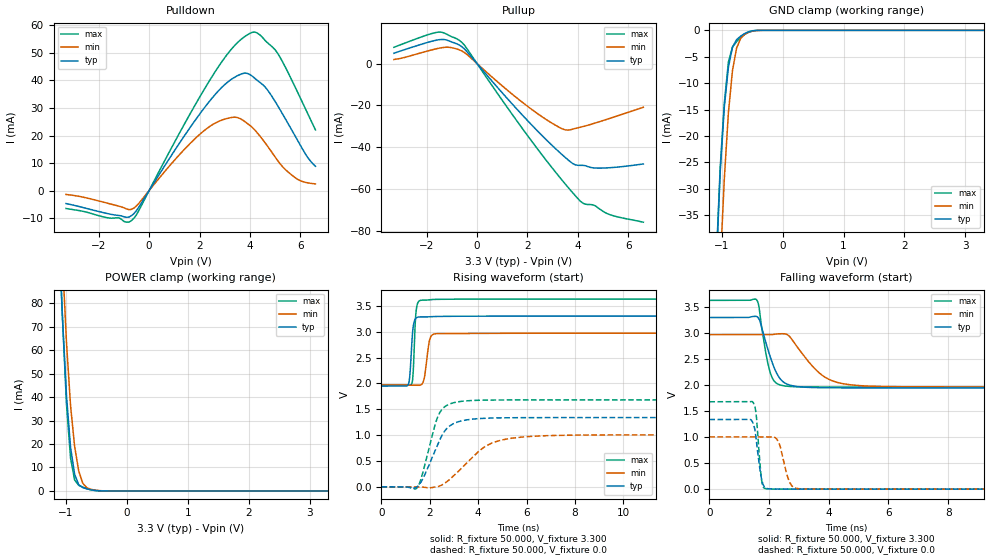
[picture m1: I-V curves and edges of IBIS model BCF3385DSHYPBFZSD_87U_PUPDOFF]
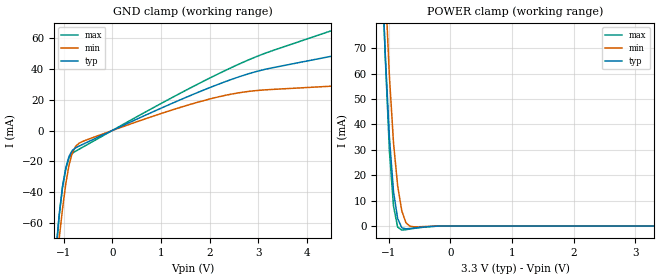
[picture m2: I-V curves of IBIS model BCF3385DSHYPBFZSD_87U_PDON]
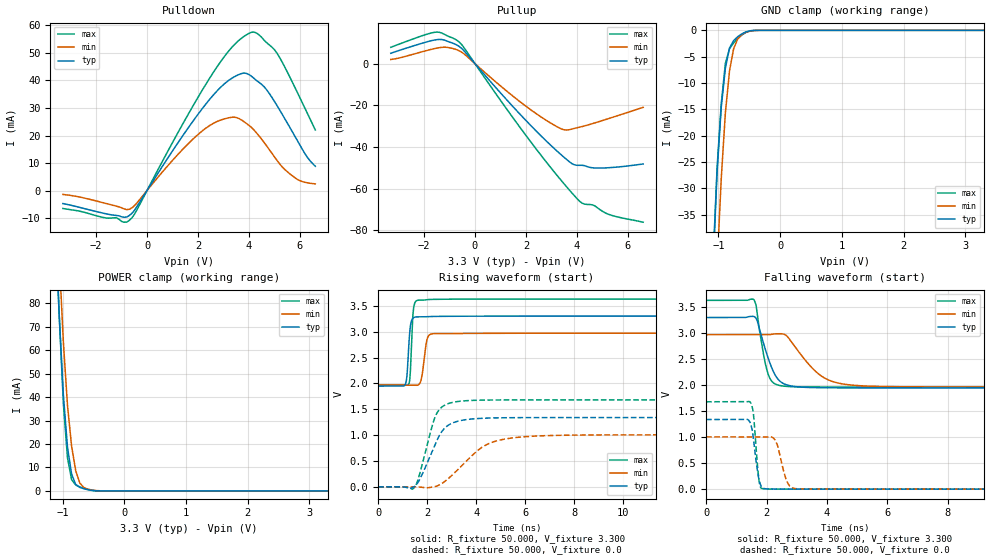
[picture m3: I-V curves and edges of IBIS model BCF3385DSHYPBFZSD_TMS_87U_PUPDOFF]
[IBIS VER]   5.0
[File Name]   am13e230pmg.ibs
[File Rev]   1.0
[Date]   February 08, 2026
[Source]   File originated at Texas Instruments
[Copyright]   (c) 2012, Texas Instruments Inc.
[Component]   am13e230pmg
[Manufacturer] Texas Instruments
[Package]
| Variable   Typ   Min   Max
   R_pkg 2.77E-01 1.56E-01 3.36E-01
   L_pkg 5.39E-09 4.33E-09 6.28E-09
   C_pkg 2.25E-14 1.68E-14 4.82E-14
[Pin]   signal_name   model_name   R_pin   L_pin   C_pin
   1   VDD   NC 3.29E-01 6.19E-09 4.32E-14
   2   PB13   BCF3385DSWHYPBFZSD_87U 3.06E-01 5.86E-09 2.08E-14
   3   PB14   BCF3385DSHYPBFZSD_87U 2.92E-01 5.63E-09 2.01E-14
   4   PB15   BCF3385DSHYPBFZSD_87U 2.81E-01 5.42E-09 1.94E-14
   5 PC16_X1   BCF3385DSHYPBFZSD_87U 2.95E-01 5.47E-09 1.88E-14
   6 PC17_X2   BCF3385DSHYPBFZSD_87U 2.91E-01 5.34E-09 1.82E-14
   7   NRST   BQ0491FSSD_XRSN_87U 2.83E-01 5.31E-09 1.75E-14
   8   PB0   BCF3385DSHYPBFZSD_87U 2.77E-01 5.15E-09 1.68E-14
   9   PB1   BCF3385DSWHYPBFZSD_87U 2.74E-01 5.11E-09 1.68E-14
   10   PB2   BCF3385DSHYPBFZSD_87U 2.76E-01 5.23E-09 1.74E-14
   11   PB3   BCF3385DSHYPBFZSD_87U 2.81E-01 5.24E-09 1.81E-14
   12   PA0   BCF3385DSWHYPBFZSD_87U 2.74E-01 5.26E-09 1.87E-14
   13   PA1   BCF3385DSHYPBFZSD_87U 2.80E-01 5.41E-09 1.94E-14
   14   PA2   BCF3385DSWHYPBFZSD_87U 2.90E-01 5.61E-09 2.01E-14
   15   VSSA   NC 1.61E-01 4.37E-09 2.30E-14
   16   VDDA   NC 1.69E-01 4.55E-09 4.78E-14
   17   PA3   BCF3385DSHYPBFZSD_87U 3.15E-01 6.06E-09 4.32E-14
   18   PA4   BCF3385DSHYPBFZSD_87U 2.94E-01 5.76E-09 2.08E-14
   19   PA5   BCF3385DSHYPBFZSD_87U 2.80E-01 5.52E-09 2.01E-14
   20   PA6   BCF3385DSHYPBFZSD_87U 2.70E-01 5.32E-09 1.94E-14
   21   PA7   BCF3385DSHYPBFZSD_87U 2.63E-01 5.16E-09 1.87E-14
   22   PB4   BCF3385DSHYPBFZSD_87U 2.61E-01 5.05E-09 1.80E-14
   23   PB5   BCF3385DSWHYPBFZSD_87U 2.63E-01 5.11E-09 1.74E-14
   24   PA16   BCF3385DSHYPBFZSD_87U 2.69E-01 5.07E-09 1.68E-14
   25   PA17   BCF3385DSHYPBFZSD_87U 2.85E-01 5.24E-09 1.69E-14
   26   PA18   BCF3385DSHYPBFZSD_87U 2.98E-01 5.47E-09 1.77E-14
   27   VREFLO   NC 3.02E-01 5.46E-09 1.83E-14
   28   VREFHI   NC 3.09E-01 5.63E-09 1.90E-14
   29   VDDA   NC 3.30E-01 5.94E-09 1.98E-14
   30   PA26   BCF3385DSHYPBFZSD_87U 2.80E-01 5.52E-09 2.01E-14
   31   VSS   NC 1.56E-01 4.33E-09 2.30E-14
   32   VDD   NC 3.10E-01 6.02E-09 4.32E-14
   33   PA27   BCF3385DSHYPBFZSD_87U 3.08E-01 5.98E-09 4.29E-14
   34   PA28   BCF3385DSHYPBFZSD_87U 2.92E-01 5.72E-09 2.07E-14
   35   PA29   BCF3385DSHYPBFZSD_87U 2.81E-01 5.51E-09 2.00E-14
   36   PA30   BCF3385DSHYPBFZSD_87U 2.74E-01 5.35E-09 1.93E-14
   37   PA31   BCF3385DSHYPBFZSD_87U 2.71E-01 5.22E-09 1.87E-14
   38   PB6   BCF3385DSHYPBFZSD_87U 2.85E-01 5.27E-09 1.81E-14
   39   PB7   BCF3385DSHYPBFZSD_87U 2.78E-01 5.25E-09 1.74E-14
   40   PB8   BCF3385DSHYPBFZSD_87U 2.79E-01 5.17E-09 1.68E-14
   41   PB9   BCF3385DSHYPBFZSD_87U 2.74E-01 5.11E-09 1.68E-14
   42   PA8   BCF3385DSHYPBFZSD_87U 2.74E-01 5.22E-09 1.74E-14
   43   PA9   BCF3385DSHYPBFZSD_87U 2.79E-01 5.22E-09 1.81E-14
   44   PA10   BCF3385DSHYPBFZSD_87U 2.87E-01 5.40E-09 1.88E-14
   45   PA11   BCF3385DSHYPBFZSD_87U 2.86E-01 5.48E-09 1.94E-14
   46   PA12  BCPF335585DSHYPBFZSD_87U 2.98E-01 5.69E-09 2.01E-14
   47   VSS   NC 3.19E-01 5.99E-09 2.09E-14
   48   VDD   NC 1.77E-01 4.63E-09 4.82E-14
   49   PA13 BCF3385DSHYPBFZSD_TMS_87U 3.36E-01 6.28E-09 4.35E-14
   50   PA14 BCF3385DSHYPBFZSD_TMS_87U 2.84E-01 5.65E-09 2.07E-14
   51   PA15  BCPF335585DSHYPBFZSD_87U 2.72E-01 5.44E-09 2.00E-14
   52   PB10   BCF3385DSHYPBFZSD_87U 2.64E-01 5.26E-09 1.93E-14
   53   PB11   BCF3385DSHYPBFZSD_87U 2.61E-01 5.13E-09 1.87E-14
   54   PB12   BCF3385DSHYPBFZSD_87U 2.61E-01 5.05E-09 1.80E-14
   55   PB18  BCPF335585DSHYPBFZSD_87U 2.64E-01 5.12E-09 1.74E-14
   56   PA19  BCPF335585DSHYPBFZSD_87U 2.66E-01 5.05E-09 1.68E-14
   57   PA20   BCF3385DSHYPBFZSD_87U 2.65E-01 5.03E-09 1.68E-14
   58   PA21   BCF3385DSHYPBFZSD_87U 2.65E-01 5.14E-09 1.74E-14
   59   PA22   BCF3385DSHYPBFZSD_87U 2.71E-01 5.14E-09 1.81E-14
   60   PA23   BCF3385DSHYPBFZSD_87U 2.80E-01 5.33E-09 1.88E-14
   61   PA24   BCF3385DSHYPBFZSD_87U 2.89E-01 5.52E-09 1.95E-14
   62   PA25   BCF3385DSHYPBFZSD_87U 3.05E-01 5.77E-09 2.03E-14
   63   VSS   NC 1.65E-01 4.43E-09 2.32E-14
   64   VDD   NC 3.23E-01 6.14E-09 4.33E-14
| End of package information
|   Component BCF3385DSHYPBFZSD_87U
[Component] BCF3385DSHYPBFZSD_87U
[Manufacturer] Texas Instruments
[Package]
| variable   typ   min   max
R_pkg   0.0   0.0   0.0
L_pkg   0.0H   0.0H   0.0H
C_pkg   0.0F   0.0F   0.0F
[Pin]  signal_name   model_name   R_pin   L_pin   C_pin
PAD   PAD   BCF3385DSHYPBFZSD_87U
VDDS   VDDS   Power
VSS   VSS   Gnd
A   A   NC
GZ   GZ   NC
[Model Selector] BCF3385DSHYPBFZSD_87U
BCF3385DSHYPBFZSD_87U_PUPDOFF PI=1 PSEL=1
BCF3385DSHYPBFZSD_87U_PDON PI=0 PSEL=0
BCF3385DSHYPBFZSD_87U_PUON PI=0 PSEL=1
|   Component BCF3385DSHYPBFZSD_TMS_87U
[Component] BCF3385DSHYPBFZSD_TMS_87U
[Manufacturer] Texas Instruments
[Package]
| variable   typ   min   max
R_pkg   0.0   0.0   0.0
L_pkg   0.0H   0.0H   0.0H
C_pkg   0.0F   0.0F   0.0F
[Pin]  signal_name   model_name   R_pin   L_pin   C_pin
PAD   PAD   BCF3385DSHYPBFZSD_TMS_87U
VDDS   VDDS   Power
VSS   VSS   Gnd
A   A   NC
GZ   GZ   NC
[Model Selector] BCF3385DSHYPBFZSD_TMS_87U
BCF3385DSHYPBFZSD_TMS_87U_PUPDOFF PI=1 PSEL=1
BCF3385DSHYPBFZSD_TMS_87U_PDON PI=0 PSEL=0
BCF3385DSHYPBFZSD_TMS_87U_PUON PI=0 PSEL=1
|   Component BCF3385DSWHYPBFZSD_87U
[Component] BCF3385DSWHYPBFZSD_87U
[Manufacturer] Texas Instruments
[Package]
| variable   typ   min   max
R_pkg   0.0   0.0   0.0
L_pkg   0.0H   0.0H   0.0H
C_pkg   0.0F   0.0F   0.0F
[Pin]  signal_name   model_name   R_pin   L_pin   C_pin
PAD   PAD   BCF3385DSWHYPBFZSD_87U
VDDS   VDDS   Power
VSS   VSS   Gnd
A   A   NC
GZ   GZ   NC
[Model Selector] BCF3385DSWHYPBFZSD_87U
BCF3385DSWHYPBFZSD_87U_PUPDOFF PI=1 PSEL=1
BCF3385DSWHYPBFZSD_87U_PDON PI=0 PSEL=0
BCF3385DSWHYPBFZSD_87U_PUON PI=0 PSEL=1
|   Component BCPF335585DSHYPBFZSD_87U
[Component] BCPF335585DSHYPBFZSD_87U
[Manufacturer] Texas Instruments
[Package]
| variable   typ   min   max
R_pkg   0.0   0.0   0.0
L_pkg   0.0H   0.0H   0.0H
C_pkg   0.0F   0.0F   0.0F
[Pin]  signal_name   model_name   R_pin   L_pin   C_pin
PAD   PAD   BCPF335585DSHYPBFZSD_87U
VDDS   VDDS   Power
VSS   VSS   Gnd
A   A   NC
GZ   GZ   NC
[Model Selector] BCPF335585DSHYPBFZSD_87U
BCPF335585DSHYPBFZSD_87U_PUPDOFF_D0 DS=0
BCPF335585DSHYPBFZSD_87U_PUPDOFF_D1 DS=1
BCPF335585DSHYPBFZSD_87U_PDON PI=0 PSEL=0
BCPF335585DSHYPBFZSD_87U_PUON PI=0 PSEL=1
|   Component BQ0491FSSD_XRSN_87U
[Component] BQ0491FSSD_XRSN_87U
[Manufacturer] Texas Instruments
[Package]
| variable   typ   min   max
R_pkg   0.0   0.0   0.0
L_pkg   0.0H   0.0H   0.0H
C_pkg   0.0F   0.0F   0.0F
[Pin]  signal_name   model_name   R_pin   L_pin   C_pin
PAD   PAD   BQ0491FSSD_XRSN_87U
VDDS   VDDS   Power
VSS   VSS   Gnd
A   A   NC
[Model Selector] BQ0491FSSD_XRSN_87U
BQ0491FSSD_XRSN_87U_PUPDOFF PI=1
BQ0491FSSD_XRSN_87U_PUPDON PI=0
| Models and submodels in the file (15): BCF3385DSHYPBFZSD_87U_PUPDOFF (I/O), BCF3385DSHYPBFZSD_87U_PDON (Input), BCF3385DSHYPBFZSD_87U_PUON (Input), BCF3385DSHYPBFZSD_TMS_87U_PUPDOFF (I/O), BCF3385DSHYPBFZSD_TMS_87U_PDON (Input), BCF3385DSHYPBFZSD_TMS_87U_PUON (Input), BCF3385DSWHYPBFZSD_87U_PUPDOFF (I/O), BCF3385DSWHYPBFZSD_87U_PDON (Input), BCF3385DSWHYPBFZSD_87U_PUON (Input), BCPF335585DSHYPBFZSD_87U_PUPDOFF_D0 (I/O), BCPF335585DSHYPBFZSD_87U_PUPDOFF_D1 (I/O), BCPF335585DSHYPBFZSD_87U_PDON (Input), BCPF335585DSHYPBFZSD_87U_PUON (Input), BQ0491FSSD_XRSN_87U_PUPDOFF (Input), BQ0491FSSD_XRSN_87U_PUPDON (Input)
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|   Model BCF3385DSHYPBFZSD_87U_PUPDOFF
[Model] BCF3385DSHYPBFZSD_87U_PUPDOFF
Model_type I/O
Polarity   Non-Inverting
Enable   Active-Low
Vinl =  0.990V
Vinh =  2.310V
Vmeas =  1.650V
C_comp   0.589pF   0.544pF   0.642pF
[Model Spec]
Vinh   2.310V   2.079V   2.541V
Vinl   0.990V   0.891V   1.089V
Vmeas   1.650V   1.485V   1.815V
[Temperature Range]   25.000   0.155k   -40.000
[Voltage Range]   3.300V   2.970V   3.630V
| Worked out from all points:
|   slope of the pulldown table from 0 to 0.495 V, typ, clamps not added: 68.5 ohm
|   slope of the pullup table from 0 to 0.495 V, typ, clamps not added: 70.6 ohm
|   GND clamp passes 1 mA (typ) near -0.67 V on its own axis
|   POWER clamp passes 1 mA (typ) near -0.67 V on its own axis
|   rising waveform, R_fixture 50.000, V_fixture 3.300: 20-80 % time 110ps typ, 165ps min, 91.9ps max; typ from 1.95 V to 3.3 V
|   rising waveform, R_fixture 50.000, V_fixture 0.0: 20-80 % time 779ps typ, 1.42ns min, 574ps max; typ from 0 V to 1.34 V
|   falling waveform, R_fixture 50.000, V_fixture 3.300: 20-80 % time 475ps typ, 935ps min, 302ps max; typ from 3.3 V to 1.95 V
|   falling waveform, R_fixture 50.000, V_fixture 0.0: 20-80 % time 180ps typ, 263ps min, 136ps max; typ from 1.34 V to 0 V
[Pulldown]
|Voltage   I(typ)   I(min)   I(max)
-3.3V     -4.738mA   -1.439mA   -6.529mA
-700mV    -9.134mA   -6.846mA   -10.9mA
-400mV    -5.894mA   -4.558mA   -7.098mA
1.4V      19.9mA     14.97mA    24.17mA
2.4V      32.5mA     23.26mA    40.01mA
3.4V      41.22mA    26.67mA    52.78mA
3.8V      42.69mA    25.06mA    56.01mA
4.1V      41.52mA    22.89mA    57.53mA
4.6V      37.66mA    17.36mA    54.58mA
5.1V      30.85mA    10.91mA    49.89mA
5.9V      18.1mA     4.028mA    35.58mA
6.6V      8.813mA    2.416mA    22.04mA
[Pullup]
|Voltage   I(typ)   I(min)   I(max)
-3.3V     4.951mA    1.968mA    7.808mA
-1.5V     11.48mA    7.414mA    15.11mA
-700mV    8.858mA    6.582mA    11.1mA
-400mV    5.719mA    4.386mA    7.142mA
2V        -27.27mA   -20.43mA   -34.44mA
3.5V      -44.98mA   -31.75mA   -57.71mA
3.9V      -48.52mA   -31.06mA   -63.34mA
4.2V      -48.76mA   -30.19mA   -66.89mA
4.6V      -49.94mA   -28.81mA   -67.71mA
4.9V      -50.09mA   -27.68mA   -69.99mA
5.4V      -49.78mA   -25.73mA   -72.89mA
6.6V      -48.1mA    -20.94mA   -76.01mA
[GND_clamp]
|Voltage   I(typ)   I(min)   I(max)
-3.3V     -1.006A    -883.4mA   -1.272A
-1.089V   -45.1mA    -63.73mA   -44.09mA
-1.022V   -26.78mA   -44.63mA   -25.9mA
-955mV    -14.49mA   -28.18mA   -13.81mA
-888mV    -7.028mA   -15.64mA   -6.005mA
-821mV    -3.189mA   -7.628mA   -3.171mA
-754mV    -1.786mA   -3.389mA   -2.151mA
-687mV    -1.097mA   -1.538mA   -1.399mA
-620mV    -601.7uA   -747.3uA   -782.8uA
-486mV    -70.11uA   -129.5uA   -99.51uA
-352mV    -1.527uA   -8.942uA   -1.719uA
3.3V      0A         0A         0A
[POWER_clamp]
|Voltage   I(typ)   I(min)   I(max)
-3.3V     1.772A     2.005A     1.902A
-1.122V   114.9mA    142.9mA    120.1mA
-1.055V   74.53mA    99.87mA    74.96mA
-988mV    40.92mA    63.48mA    37.22mA
-921mV    18.54mA    36.45mA    14.02mA
-854mV    7.11mA     18.97mA    4.658mA
-787mV    2.624mA    8.509mA    2.397mA
-720mV    1.421mA    3.258mA    1.612mA
-653mV    867.1uA    1.356mA    992.6uA
-586mV    464.5uA    677.9uA    496.7uA
-385mV    10.92uA    45.23uA    6.451uA
3.3V      0A         0A         0A
[Ramp]
| variable   typ   min   max
dV/dt_r   0.803/0.779n   0.603/1.418n   1.008/0.574n
dV/dt_f   0.812/0.475n   0.602/0.935n   1.000/0.302n
R_load = 50.000
[Rising Waveform]
R_fixture= 50.000
V_fixture= 3.300
V_fixture_min= 2.970
V_fixture_max= 3.630
|time   V(typ)   V(min)   V(max)
0s        1.947V     1.966V     1.964V
1.09ns    1.964V     1.966V     1.965V
1.173ns   2.148V     1.966V     1.963V
1.247ns   2.706V     1.966V     1.983V
1.305ns   3.069V     1.966V     2.16V
1.431ns   3.263V     1.965V     3.391V
1.642ns   3.286V     1.973V     3.607V
1.999ns   3.289V     2.857V     3.619V
2.245ns   3.294V     2.96V      3.624V
25ns      3.3V       2.97V      3.63V
[Rising Waveform]
R_fixture= 50.000
V_fixture= 0.0
V_fixture_min= 0.0
V_fixture_max= 0.0
|time   V(typ)   V(min)   V(max)
0s        1.247uV    1.099uV    1.11uV
1.478ns   2.237mV    651.3uV    -15.09mV
1.668ns   120.2mV    -3.627mV   205.2mV
2.197ns   681.3mV    -6.221mV   1.167V
2.376ns   875.6mV    11.23mV    1.405V
2.726ns   1.14V      107.1mV    1.581V
3.219ns   1.264V     317.4mV    1.648V
4.459ns   1.329V     823.6mV    1.677V
6.109ns   1.338V     973.1mV    1.68V
25ns      1.339V     1.005V     1.68V
[Falling Waveform]
R_fixture= 50.000
V_fixture= 3.300
V_fixture_min= 2.970
V_fixture_max= 3.630
|time   V(typ)   V(min)   V(max)
0s        3.3V       2.97V      3.63V
1.579ns   3.32V      2.97V      3.643V
1.657ns   3.281V     2.97V      3.525V
1.851ns   2.905V     2.97V      2.753V
2.055ns   2.52V      2.97V      2.215V
2.3ns     2.183V     2.986V     2.02V
2.568ns   2.03V      2.981V     1.982V
3.798ns   1.95V      2.183V     1.964V
4.918ns   1.947V     1.996V     1.964V
25ns      1.947V     1.966V     1.964V
[Falling Waveform]
R_fixture= 50.000
V_fixture= 0.0
V_fixture_min= 0.0
V_fixture_max= 0.0
|time   V(typ)   V(min)   V(max)
0s        1.339V     1.005V     1.68V
1.474ns   1.257V     1.005V     1.662V
1.571ns   953.8mV    1.005V     1.426V
1.696ns   371.1mV    1.005V     488.6mV
1.758ns   172.9mV    1.005V     144.9mV
1.921ns   14.01mV    1.005V     7.462mV
2.281ns   1.937mV    944.6mV    1.495mV
2.686ns   766.7uV    139.7mV    436.8uV
3.029ns   353.8uV    7.281mV    145.5uV
25ns      332.8nV    598.9nV    336.5nV
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|   Model BCF3385DSHYPBFZSD_87U_PDON
[Model] BCF3385DSHYPBFZSD_87U_PDON
Model_type Input
Polarity   Non-Inverting
Enable   Active-High
Vinl =  0.990V
Vinh =  2.310V
C_comp   0.593pF   0.545pF   0.644pF
[Model Spec]
Vinh   2.310V   2.079V   2.541V
Vinl   0.990V   0.891V   1.089V
[Temperature Range]   25.000   0.155k   -40.000
[Voltage Range]   3.300V   2.970V   3.630V
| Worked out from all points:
|   GND clamp passes 1 mA (typ) near -0.07 V on its own axis
|   POWER clamp passes 1 mA (typ) near -0.67 V on its own axis
[GND_clamp]
|Voltage   I(typ)   I(min)   I(max)
-3.3V     -1.011A    -884.9mA   -1.28A
-1.156V   -76.88mA   -90.37mA   -80.57mA
-1.089V   -54.34mA   -69.73mA   -54.73mA
-1.022V   -36.25mA   -50.83mA   -37.1mA
-955mV    -24.19mA   -34.63mA   -25.16mA
-888mV    -16.76mA   -22.37mA   -17.58mA
-821mV    -12.88mA   -14.56mA   -14.76mA
-754mV    -11.23mA   -10.35mA   -13.41mA
1.189V    17.02mA    12.89mA    20.64mA
2.328V    31.68mA    22.8mA     38.93mA
3.266V    40.44mA    26.55mA    51.4mA
6.6V      60.98mA    32.35mA    86.96mA
[POWER_clamp]
|Voltage   I(typ)   I(min)   I(max)
-3.3V     1.722A     1.973A     1.84A
-1.122V   107.2mA    137.2mA    110.5mA
-1.055V   67.72mA    94.79mA    66.44mA
-988mV    34.94mA    59.05mA    29.78mA
-921mV    13.45mA    32.66mA    7.761mA
-854mV    2.926mA    15.82mA    -428.8uA
-787mV    -691.9uA   5.965mA    -1.61mA
-720mV    -1.106mA   1.289mA    -1.422mA
-653mV    -960.7uA   -93.94uA   -1.168mA
-586mV    -772.5uA   -324.4uA   -929.9uA
-117mV    0A         0A         0A
3.3V      0A         0A         0A
|   Model BCF3385DSHYPBFZSD_TMS_87U_PUPDOFF
[Model] BCF3385DSHYPBFZSD_TMS_87U_PUPDOFF
Model_type I/O
Polarity   Non-Inverting
Enable   Active-Low
Vinl =  0.990V
Vinh =  2.310V
Vmeas =  1.650V
C_comp   0.559pF   0.509pF   0.619pF
[Model Spec]
Vinh   2.310V   2.079V   2.541V
Vinl   0.990V   0.891V   1.089V
Vmeas   1.650V   1.485V   1.815V
[Temperature Range]   25.000   0.155k   -40.000
[Voltage Range]   3.300V   2.970V   3.630V
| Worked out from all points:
|   slope of the pulldown table from 0 to 0.495 V, typ, clamps not added: 68.5 ohm
|   slope of the pullup table from 0 to 0.495 V, typ, clamps not added: 70.6 ohm
|   GND clamp passes 1 mA (typ) near -0.66 V on its own axis
|   POWER clamp passes 1 mA (typ) near -0.66 V on its own axis
|   rising waveform, R_fixture 50.000, V_fixture 3.300: 20-80 % time 110ps typ, 163ps min, 90.4ps max; typ from 1.95 V to 3.3 V
|   rising waveform, R_fixture 50.000, V_fixture 0.0: 20-80 % time 779ps typ, 1.42ns min, 574ps max; typ from 0 V to 1.34 V
|   falling waveform, R_fixture 50.000, V_fixture 3.300: 20-80 % time 474ps typ, 934ps min, 300ps max; typ from 3.3 V to 1.95 V
|   falling waveform, R_fixture 50.000, V_fixture 0.0: 20-80 % time 179ps typ, 262ps min, 135ps max; typ from 1.34 V to 0 V
[Pulldown]
|Voltage   I(typ)   I(min)   I(max)
-3.3V     -4.742mA   -1.441mA   -6.54mA
-700mV    -9.13mA    -6.846mA   -10.89mA
-400mV    -5.894mA   -4.558mA   -7.098mA
1.4V      19.9mA     14.97mA    24.17mA
2.4V      32.5mA     23.27mA    40.01mA
3.4V      41.22mA    26.67mA    52.78mA
3.8V      42.69mA    25.06mA    56.01mA
4.1V      41.53mA    22.89mA    57.54mA
4.6V      37.66mA    17.36mA    54.59mA
5.1V      30.85mA    10.91mA    49.89mA
5.9V      18.1mA     4.028mA    35.58mA
6.6V      8.814mA    2.416mA    22.04mA
[Pullup]
|Voltage   I(typ)   I(min)   I(max)
-3.3V     4.951mA    1.968mA    7.808mA
-1.5V     11.48mA    7.414mA    15.11mA
-700mV    8.857mA    6.582mA    11.1mA
-400mV    5.719mA    4.386mA    7.142mA
2V        -27.27mA   -20.43mA   -34.44mA
3.5V      -44.98mA   -31.75mA   -57.71mA
3.9V      -48.52mA   -31.06mA   -63.34mA
4.2V      -48.76mA   -30.19mA   -66.89mA
4.6V      -49.94mA   -28.82mA   -67.71mA
4.9V      -50.09mA   -27.69mA   -69.99mA
5.4V      -49.79mA   -25.74mA   -72.9mA
6.6V      -48.13mA   -20.97mA   -76.04mA
[GND_clamp]
|Voltage   I(typ)   I(min)   I(max)
-3.3V     -1.006A    -883.6mA   -1.273A
-1.089V   -45.2mA    -63.83mA   -44.22mA
-1.022V   -26.88mA   -44.72mA   -26.06mA
-955mV    -14.62mA   -28.27mA   -14.02mA
-888mV    -7.183mA   -15.73mA   -6.291mA
-821mV    -3.37mA    -7.718mA   -3.478mA
-754mV    -1.948mA   -3.475mA   -2.39mA
-687mV    -1.208mA   -1.613mA   -1.554mA
-620mV    -663.5uA   -801.3uA   -867.2uA
-553mV    -281.3uA   -375.3uA   -374.8uA
-352mV    -1.803uA   -10.08uA   -2.106uA
3.3V      0A         0A         0A
[POWER_clamp]
|Voltage   I(typ)   I(min)   I(max)
-3.3V     1.772A     2.005A     1.902A
-1.122V   114.9mA    143mA      120.1mA
-1.055V   74.57mA    99.89mA    75.01mA
-988mV    40.96mA    63.5mA     37.28mA
-921mV    18.59mA    36.47mA    14.09mA
-854mV    7.17mA     19mA       4.772mA
-787mV    2.703mA    8.539mA    2.533mA
-720mV    1.495mA    3.291mA    1.714mA
-653mV    916.7uA    1.391mA    1.057mA
-586mV    491.6uA    704.5uA    530.7uA
-385mV    11.77uA    47.43uA    7.131uA
3.3V      0A         0A         0A
[Ramp]
| variable   typ   min   max
dV/dt_r   0.803/0.779n   0.603/1.418n   1.008/0.574n
dV/dt_f   0.812/0.474n   0.602/0.934n   1.000/0.300n
R_load = 50.000
[Rising Waveform]
R_fixture= 50.000
V_fixture= 3.300
V_fixture_min= 2.970
V_fixture_max= 3.630
|time   V(typ)   V(min)   V(max)
0s        1.947V     1.966V     1.964V
1.089ns   1.963V     1.966V     1.965V
1.174ns   2.154V     1.966V     1.963V
1.25ns    2.736V     1.966V     1.986V
1.309ns   3.092V     1.966V     2.19V
1.432ns   3.267V     1.965V     3.41V
1.63ns    3.286V     1.97V      3.608V
1.998ns   3.289V     2.859V     3.619V
2.246ns   3.294V     2.96V      3.624V
25ns      3.3V       2.97V      3.63V
[Rising Waveform]
R_fixture= 50.000
V_fixture= 0.0
V_fixture_min= 0.0
V_fixture_max= 0.0
|time   V(typ)   V(min)   V(max)
0s        1.248uV    1.099uV    1.113uV
1.474ns   963.4uV    647.9uV    -16.94mV
1.665ns   117.8mV    -3.519mV   201.9mV
2.194ns   678.4mV    -6.423mV   1.163V
2.373ns   872.9mV    10.75mV    1.404V
2.728ns   1.141V     107.7mV    1.582V
3.226ns   1.265V     320.4mV    1.648V
4.455ns   1.329V     822.7mV    1.677V
6.105ns   1.338V     973mV      1.68V
25ns      1.339V     1.005V     1.68V
[Falling Waveform]
R_fixture= 50.000
V_fixture= 3.300
V_fixture_min= 2.970
V_fixture_max= 3.630
|time   V(typ)   V(min)   V(max)
0s        3.3V       2.97V      3.63V
1.579ns   3.32V      2.97V      3.643V
1.657ns   3.281V     2.97V      3.526V
1.867ns   2.872V     2.97V      2.699V
2.062ns   2.507V     2.97V      2.198V
2.304ns   2.177V     2.986V     2.018V
2.574ns   2.027V     2.98V      1.981V
3.796ns   1.95V      2.183V     1.964V
4.916ns   1.947V     1.996V     1.964V
25ns      1.947V     1.966V     1.964V
[Falling Waveform]
R_fixture= 50.000
V_fixture= 0.0
V_fixture_min= 0.0
V_fixture_max= 0.0
|time   V(typ)   V(min)   V(max)
0s        1.339V     1.005V     1.68V
1.474ns   1.257V     1.005V     1.662V
1.572ns   949.6mV    1.005V     1.421V
1.691ns   385.6mV    1.005V     515.2mV
1.758ns   167.9mV    1.005V     136.6mV
1.896ns   16.86mV    1.005V     7.503mV
2.28ns    1.832mV    945.7mV    1.454mV
2.695ns   731.9uV    125.9mV    409.2uV
3.023ns   346.7uV    6.842mV    137.9uV
25ns      18.51nV    163.2nV    42.26nV
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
